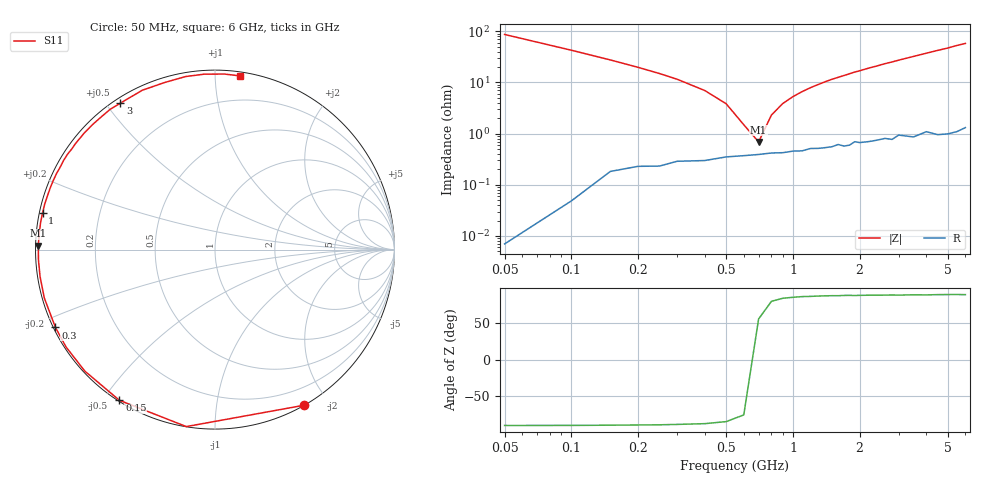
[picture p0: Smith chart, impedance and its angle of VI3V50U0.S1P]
! Infineon Technologies  Discrete & RF Semiconductors
! BB 804
! Si Tuning Diode in SOT23
! VR = 3.5 V
! S-Parameters:  July  1999
# GHz  S  MA  R  50
!  f  S11
! GHz  MAG  ANG
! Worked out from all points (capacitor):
!   34 points, 50 MHz to 6 GHz, reference 50 ohm
!   read as one part to ground: C = 36.6 pF near 50 MHz
!   lowest |Z| = 689 mohm at 700 MHz (marker M1)
!   series resonance near 671.7 MHz, so ESL is about 1.5 nH
!   S11 on the Smith chart (normalised r, x): 50 MHz: 0.00, -1.73; 150 MHz: 0.00, -0.55; 300 MHz: 0.01, -0.23; 1 GHz: 0.01, +0.11; 3 GHz: 0.02, +0.54; 6 GHz: 0.03, +1.15
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0.05  0.9999 -60.1
0.1  0.9989 -99.2
0.15  0.9944 -122.4
0.2  0.9921 -137.0
0.25  0.9915 -146.8
0.3  0.9891 -154.0
0.4  0.9884 -164.2
0.5  0.9862 -171.3
0.6  0.9853 -176.7
0.7  0.9845 178.7
0.8  0.9835 174.8
1  0.9822 168.0
1.3  0.9803 159.4
1.5  0.9792 154.1
1.6  0.9772 151.8
1.7  0.979 149.5
1.9  0.9751 144.7
2.2  0.9759 138.3
2.4  0.975 134.4
2.6  0.9738 130.2
2.8  0.9757 126.7
3  0.9716 122.9
3.5  0.976 114.5
4  0.9723 106.7
4.5  0.978 99.6
5  0.9793 93.5
5.5  0.9795 86.9
6  0.9778 81.8
